(* Logix 5000 AddOnInstructionDefinition export; software revision 16.04 *)

TYPE AKD_Status :   // All connections to the drive ethernet module are established and data is successfully transferring.
STRUCT
   Profile_In_Progress : BOOL;   // Profile Move In Progress
   Block_In_Execution : BOOL;   // Block In Execution
   On_Target_Position : BOOL;   // On Target Position (1=Current Position Equals Last Target Position)
   General_Fault : BOOL;   // General Fault
   Current_Direction : BOOL;   // Current Motor Direction (0=Reverse, 1=Forward)
   Home_Level : BOOL;   // Level of Home Input
   Reg_Level : BOOL;   // Level of Registration Input
   Enable : BOOL;   // State of Enable Output
   Fault_Input_Fault : BOOL;   // Fault Input Active
   Fwd_Limit : BOOL;   // Forward Input Active
   Rev_Limit : BOOL;   // Reverse Input Active
   Positive_Limit : BOOL;   // Positive Software Limit Exceeded
   Negative_Limit : BOOL;   // Negative Software Limit Exceeded
   FE_Fault : BOOL;   // Following Error Fault
   Block_Fault : BOOL;   // Block Execution Fault
   Load_Complete : BOOL;   // Command Message Successfully Loaded
END_STRUCT
END_TYPE

TYPE AKD_Axis :   // Axis Data:
STRUCT
   Control : AKD_Control;   // Control bits to send to the drive
   Status : AKD_Status;   // Status bits received from the drive
   Input : AB:ETHERNET_MODULE_SINT_64Bytes:I:0;   // Data from the drive
   Output : AB:ETHERNET_MODULE_SINT_64Bytes:O:0;   // Data to the drive
   ResponseMsgType : SINT;   // Response type contained in latest IO response from drive. Used to check for errors
   CommandTimeout : INT;   // Time to allow for command response from drive. Dependent on scan rate and communicaiton rate
   PositionFeedback : DINT;   // Actual Position Value
   VelocityFeedback : DINT;   // Actual Velocity Value
END_STRUCT
END_TYPE

TYPE AKD_Control :   // Send Explicit Message
STRUCT
   Load_Data_Start_Profile : BOOL;   // Load Command Data / Start Profile Move
   Start_Block : BOOL;   // Execute Command block or block chain
   Incremental : BOOL;   // Incremental Position (0=Absolute, 1=Incremental)
   Direction : BOOL;   // Direction in Velocity Mode (0=Reverse, 1=Forward)
   Smooth_Stop : BOOL;   // Smooth / Controlled Stop w/ Deceleration
   Hard_Stop : BOOL;   // Hard / Immediate Stop
   Reg_Arm : BOOL;   // Arm the Registration Input
   Enable : BOOL;   // Enable Output
END_STRUCT
END_TYPE

ADD_ON_INSTRUCTION AKD_Set_Attribute   (* revision 2.1, ExecutePrescan, ExecuteEnableInFalse *)
// Set Position Controller Attribute
// Revision note:
// Don't error if Command_Timeout preset is 0
VAR_OUTPUT
   DN : BOOL; {visible}   // Command Successful
   ER : BOOL; {visible}   // Error
END_VAR
VAR_IN_OUT
   Axis : AKD_Axis; {required}
END_VAR
VAR_INPUT
   Attribute_Number : INT; {visible}   // Attribute Number (see help for options)
   Attribute_Value : DINT; {required}   // Attribute Value
END_VAR
VAR
   Command_Timeout : TIMER;   // Timeout Timer
   Command_Message_Type : SINT;   // Command Message Type
   Command_Axis_Number : SINT;   // Command Axis Number
   Step : SINT;
   Command_Bytes : SINT[8];
   OS_LoadStart : BOOL;
END_VAR

ROUTINE EnableInFalse   (* ladder *)
// EnableIn_False
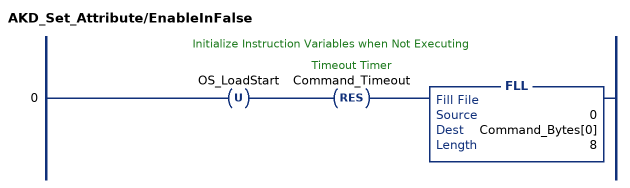
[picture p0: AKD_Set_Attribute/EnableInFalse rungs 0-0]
   // Initialize Instruction Variables when Not Executing
   0: OTU(OS_LoadStart)RES(Command_Timeout)FLL(0,Command_Bytes[0],8);
END_ROUTINE

ROUTINE Logic   (* ladder *)
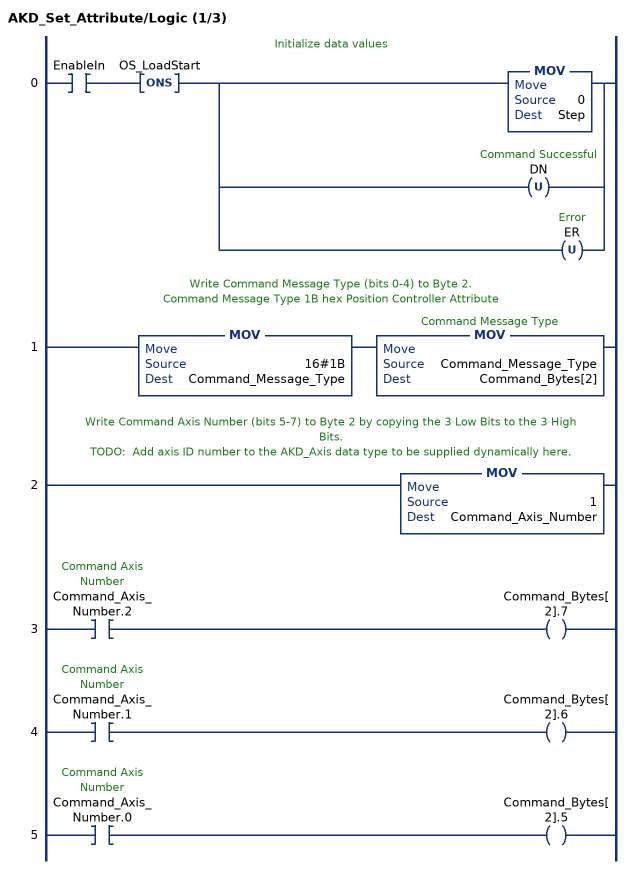
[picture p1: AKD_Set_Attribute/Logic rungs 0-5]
   // Initialize data values
   0: XIC(EnableIn)ONS(OS_LoadStart)[MOV(0,Step) ,OTU(DN) ,OTU(ER) ];
   // Write Command Message Type (bits 0-4) to Byte 2.
   // Command Message Type 1B hex Position Controller Attribute
   1: MOV(16#1B,Command_Message_Type)MOV(Command_Message_Type,Command_Bytes[2]);
   // Write Command Axis Number (bits 5-7) to Byte 2 by copying the 3 Low Bits to the 3 High Bits.
   // TODO:  Add axis ID number to the AKD_Axis data type to be supplied dynamically here.
   2: MOV(1,Command_Axis_Number);
   3: XIC(Command_Axis_Number.2)OTE(Command_Bytes[2].7);
   4: XIC(Command_Axis_Number.1)OTE(Command_Bytes[2].6);
   5: XIC(Command_Axis_Number.0)OTE(Command_Bytes[2].5);
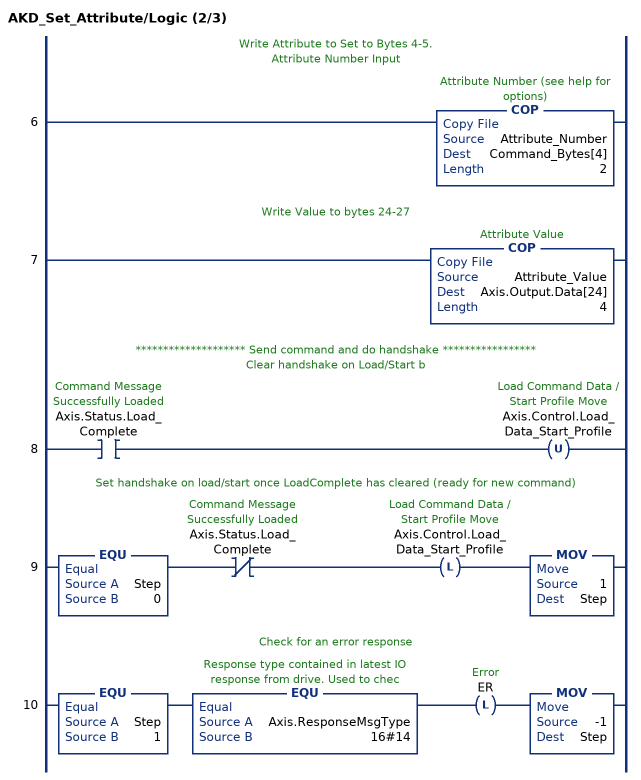
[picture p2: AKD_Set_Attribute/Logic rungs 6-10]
   // Write Attribute to Set to Bytes 4-5.
   // Attribute Number Input
   6: COP(Attribute_Number,Command_Bytes[4],2);
   // Write Value to bytes 24-27
   7: COP(Attribute_Value,Axis.Output.Data[24],4);
   // ******************** Send command and do handshake *****************
   // Clear handshake on Load/Start b
   8: XIC(Axis.Status.Load_Complete)OTU(Axis.Control.Load_Data_Start_Profile);
   // Set handshake on load/start once LoadComplete has cleared (ready for new command)
   9: EQU(Step,0)XIO(Axis.Status.Load_Complete)OTL(Axis.Control.Load_Data_Start_Profile)MOV(1,Step);
   // Check for an error response
   10: EQU(Step,1)EQU(Axis.ResponseMsgType,16#14)OTL(ER)MOV(-1,Step);
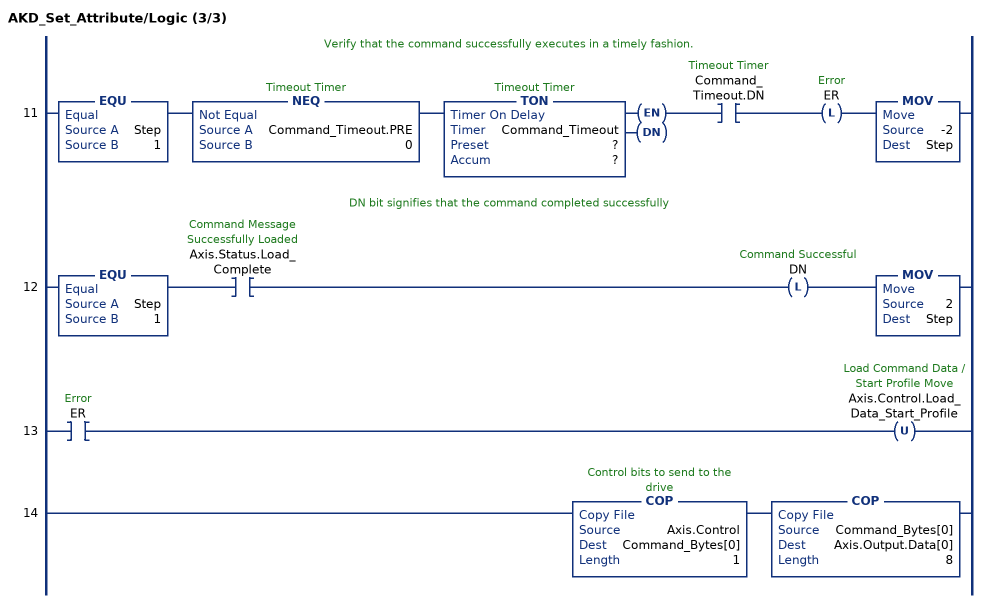
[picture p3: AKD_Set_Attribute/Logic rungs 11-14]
   // Verify that the command successfully executes in a timely fashion.
   11: EQU(Step,1)NEQ(Command_Timeout.PRE,0)TON(Command_Timeout,?,?)XIC(Command_Timeout.DN)OTL(ER)MOV(-2,Step);
   // DN bit signifies that the command completed successfully
   12: EQU(Step,1)XIC(Axis.Status.Load_Complete)OTL(DN)MOV(2,Step);
   13: XIC(ER)OTU(Axis.Control.Load_Data_Start_Profile);
   14: COP(Axis.Control,Command_Bytes[0],1)COP(Command_Bytes[0],Axis.Output.Data[0],8);
END_ROUTINE

ROUTINE Prescan   (* ladder *)
// Prescan
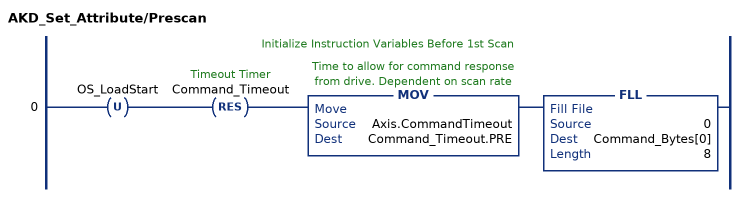
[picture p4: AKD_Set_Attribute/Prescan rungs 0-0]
   // Initialize Instruction Variables Before 1st Scan
   0: OTU(OS_LoadStart)RES(Command_Timeout)MOV(Axis.CommandTimeout,Command_Timeout.PRE)FLL(0,Command_Bytes[0],8);
END_ROUTINE
END_ADD_ON_INSTRUCTION

ADD_ON_INSTRUCTION AKD_Set_Home_Mode   (* revision 2.0, ExecutePrescan, ExecuteEnableInFalse *)
// Set Homing Mode
VAR_OUTPUT
   DN : BOOL; {visible}   // Command Successful
   ER : BOOL; {visible}   // Error
END_VAR
VAR_IN_OUT
   Axis : AKD_Axis; {required}
END_VAR
VAR_INPUT
   Mode : SINT; {required}   // Home Mode:
END_VAR
VAR
   Command_Bytes : SINT[8];
   Step : DINT;
   Set_Attribute : AKD_Set_Attribute;
END_VAR

ROUTINE EnableInFalse   (* ladder *)
// EnableIn_False
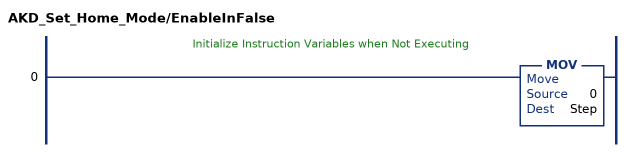
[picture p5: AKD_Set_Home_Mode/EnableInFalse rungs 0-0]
   // Initialize Instruction Variables when Not Executing
   0: MOV(0,Step);
END_ROUTINE

ROUTINE Logic   (* ladder *)
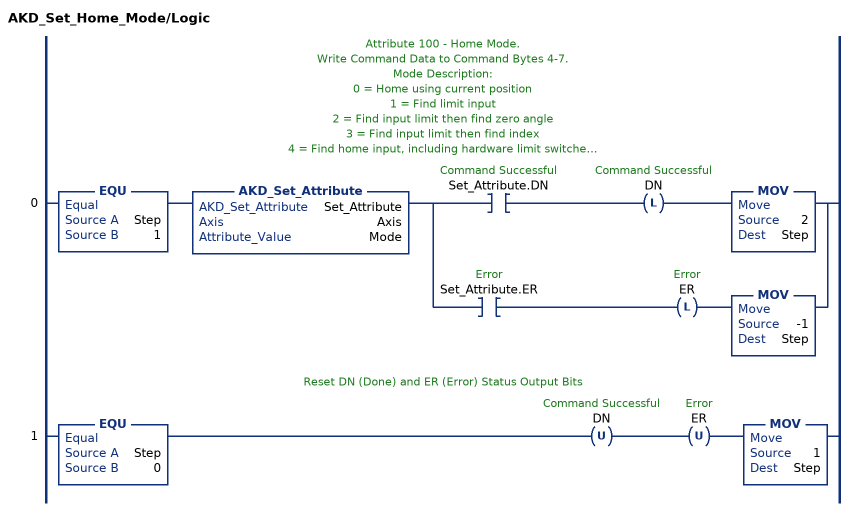
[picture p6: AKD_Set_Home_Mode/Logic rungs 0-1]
   // Attribute 100 - Home Mode.
   // Write Command Data to Command Bytes 4-7.
   // Mode Description:
   // 0 = Home using current position
   // 1 = Find limit input
   // 2 = Find input limit then find zero angle
   // 3 = Find input limit then find index
   // 4 = Find home input, including hardware limit switches
   // 5 = Find home input then find zero angle, including hardware limit switches
   // 6 = Find home input then find index, including hardware limit switches.
   // 7 = Find zero angle
   // 8 = Move until position error exceeded
   // 9 = Move until position error exceeded, then find zero angle
   // 10 = Move until position error exceeded, then find index
   // 11 = Find index signal, without any precondition
   // 12 = Homing to a home-switch, including mechanical stop detection
   0: EQU(Step,1)AKD_Set_Attribute(Set_Attribute,Axis,Mode)[XIC(Set_Attribute.DN) OTL(DN) MOV(2,Step) ,XIC(Set_Attribute.ER) OTL(ER) MOV(-1,Step) ];
   // Reset DN (Done) and ER (Error) Status Output Bits
   1: EQU(Step,0)OTU(DN)OTU(ER)MOV(1,Step);
END_ROUTINE

ROUTINE Prescan   (* ladder *)
// Prescan
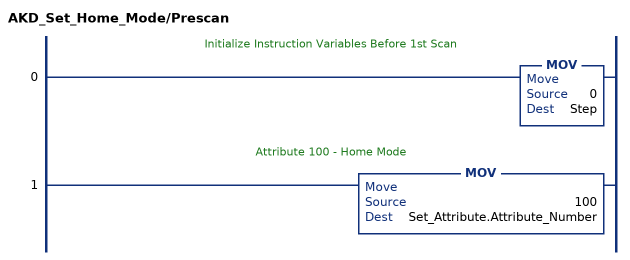
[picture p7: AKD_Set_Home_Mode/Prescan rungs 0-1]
   // Initialize Instruction Variables Before 1st Scan
   0: MOV(0,Step);
   // Attribute 100 - Home Mode
   1: MOV(100,Set_Attribute.Attribute_Number);
END_ROUTINE
END_ADD_ON_INSTRUCTION
